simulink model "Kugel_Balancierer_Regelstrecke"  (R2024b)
settings: Solver=VariableStepAuto  StartTime=0.0  StopTime=10.0  RelTol=1e-3

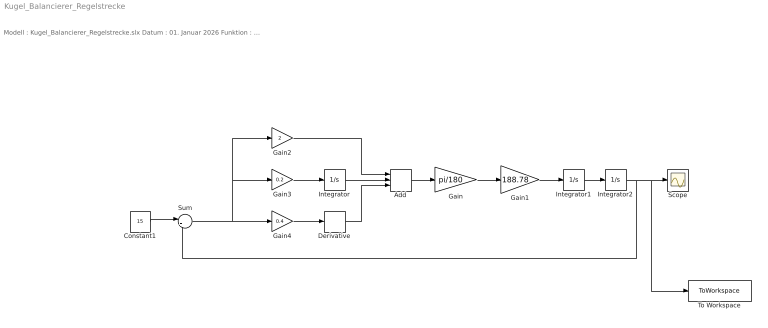
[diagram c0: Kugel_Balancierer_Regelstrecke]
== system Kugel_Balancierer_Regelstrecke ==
  note: Modell : Kugel_Balancierer_Regelstrecke.slx Datum : 01. Januar 2026 Funktion : Dieses Modell simuliert den Kugel-Balancierer. Ein PID Regler regelt das System mit der berechneten Übertragungsfunktion des realen Kugel-Balancierers. Req. Toolbox : Autor : Kilian Engelhardt, Daniel Block Bemerkung : Getestet Letzte Änderung : 01. Jan 2026
  Add : Sum  Inputs=+++
  Constant1 : Constant  Value=15
  Derivative : Derivative
  Gain : Gain  Gain=pi/180
  Gain1 : Gain  Gain=188.78
  Gain2 : Gain  Gain=2
  Gain3 : Gain  Gain=0.2
  Gain4 : Gain  Gain=0.4
  Integrator : Integrator
  Integrator1 : Integrator
  Integrator2 : Integrator
  Scope : Scope
  Sum : Sum  Inputs=|+-
  To Workspace : ToWorkspace  VariableName=regler  SaveFormat=Timeseries  SampleTime=-1
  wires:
  Constant1/1 -> Sum/1
  Sum/1 -> Gain4/1, Gain2/1, Gain3/1
  Gain3/1 -> Integrator/1
  Gain4/1 -> Derivative/1
  Gain2/1 -> Add/1
  Integrator/1 -> Add/2
  Derivative/1 -> Add/3
  Add/1 -> Gain/1
  Integrator1/1 -> Integrator2/1
  Gain/1 -> Gain1/1
  Gain1/1 -> Integrator1/1
  Integrator2/1 -> To Workspace/1, Scope/1, Sum/2
